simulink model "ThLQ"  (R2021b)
settings: Solver=VariableStepAuto  StartTime=0.0  StopTime=timeWaypoints(end)-0.2  RelTol=1e-3
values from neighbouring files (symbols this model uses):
  a = 0.27    [CompareGazeboSimulink.m]    (also in RobotModel.m)
  b = 0.31    [CompareGazeboSimulink.m]    (also in RobotModel.m)
  D = abs(a-b)    [RobotModel.m]
  distAng = 0    [RobotModel.m]
  distVel = 0    [RobotModel.m]
  fro = 0.02    [CompareGazeboSimulink.m]    (also in RobotModel.m)
  fsl = 0.8    [CompareGazeboSimulink.m]    (also in RobotModel.m)
  fsly = 0.8    [CompareGazeboSimulink.m]    (also in RobotModel.m)
  I = (1/12)*m*((2*t)^2 + 0.12^2) + 1.5    (= 2.384)    [CompareGazeboSimulink.m]    (also in RobotModel.m = 0.866666666667)
  k = 1    [RobotModel.m]
  ko = 0    [CompareGazeboSimulink.m]    (also in RobotModel.m = 0.25)
  kt = 0.58    [CompareGazeboSimulink.m]    (also in RobotModel.m)
  kx = 0.5    [RobotModel.m]
  ky = 0.5    [RobotModel.m]
  lx = 0.15    [RobotModel.m]
  ly = 0.15    [RobotModel.m]
  m = 51    [CompareGazeboSimulink.m]    (also in RobotModel.m = 50)
  mdy = 10    [CompareGazeboSimulink.m]    (also in RobotModel.m)
  mst = 10    [CompareGazeboSimulink.m]    (also in RobotModel.m)
  Q = [1 0    [RobotModel.m]
  r = 0.19    [CompareGazeboSimulink.m]    (also in RobotModel.m)
  R = [0.01 0    [RobotModel.m]
  T_vel_variance = 0.0005    [RobotModel.m]
  Th0 = 0    [CompareGazeboSimulink.m]    (also in RobotModel.m = 0.9714)
  Th_vel0 = 0    [CompareGazeboSimulink.m]    (also in RobotModel.m)
  timeWaypoints = [0, 3, 7.5, 10.5, 13.5, 18, 20.5]    [RobotModel.m]
  Ts = 0.01    [CompareGazeboSimulink.m]    (also in RobotModel.m = 0.05)
  waypoints = [0 5; 4 9; 8 1; 12 5; 8 9; 4 1; 0 5]    [CubicSpline.m]    (also in RobotModel.m = [0 2.5; 2 4.5; 4 0.5; 6 2.5; 4 4.5; 2 0.5; 0 2.5])
  X0 = 0    [CompareGazeboSimulink.m]    (also in RobotModel.m)
  x_vel0 = 0    [CompareGazeboSimulink.m]    (also in RobotModel.m)
  x_vel_variance = 0.0005    [RobotModel.m]
  Y0 = 0    [CompareGazeboSimulink.m]    (also in RobotModel.m = 2.5)
libraries: mobileRoboticsLib x1

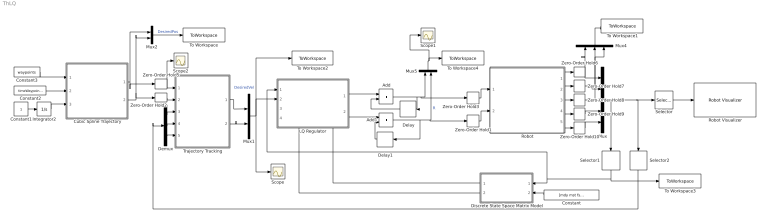
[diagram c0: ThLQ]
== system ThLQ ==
  Add : Sum
  Add1 : Sum
  Constant : Constant  Value=[mdy mst fsly r t a b m I Ts k]
  Constant1 : Constant
  Constant2 : Constant  Value=timeWaypoints
  Constant3 : Constant  Value=waypoints
  Cubic Spline Trajectory : MATLAB Function  TreatAsAtomicUnit=on
  Delay : Delay  DelayLength=1
  Delay1 : Delay  DelayLength=1
  Demux : Demux  Outputs=3
  Discrete State Space Matrix Model : MATLAB Function  TreatAsAtomicUnit=on
  Integrator2 : Integrator
  LQ Regulator : Subsystem
  Mux : Mux  Inputs=5
  Mux1 : Mux  Inputs=2
  Mux2 : Mux  Inputs=2
  Mux4 : Mux  Inputs=3
  Mux5 : Mux  Inputs=2
  Robot : Subsystem
  Robot Visualizer : mobileRoboticsLib/Environments/Robot Visualizer  Commented=on  robotRadius=0.3  showTrajectory=on  hasWaypoints=off  hasLidar=off  sensorOffset=[ 0, 0 ]  scanAngles=[ -pi/4, 0, pi/4 ]  hasObjDetector=off  objDetectorOffset=[ 0, 0 ]  objDetectorAngle=0  objDetectorFOV=pi/4  objDetectorMaxRange=5  objectColors=[ 1, 0, 0; 0, 1, 0; 0, 0, 1 ]  objectMarkers=s
  Scope : Scope
  Scope1 : Scope
  Scope2 : Scope
  Selector : Selector  InputPortWidth=5  IndexOptions=Index vector (dialog)  Indices=[1 2 3]  OutputSizes=1
  Selector1 : Selector  InputPortWidth=5  IndexOptions=Index vector (dialog)  Indices=[4 5]  OutputSizes=1
  Selector2 : Selector  InputPortWidth=5  IndexOptions=Index vector (dialog)  Indices=[1 2 3]  OutputSizes=1
  To Workspace : ToWorkspace  VariableName=desiredPos  SaveFormat=Timeseries  SampleTime=-1
  To Workspace1 : ToWorkspace  VariableName=ActualPos  SaveFormat=Timeseries  SampleTime=-1
  To Workspace2 : ToWorkspace  VariableName=DesiredVel  SaveFormat=Timeseries  SampleTime=-1
  To Workspace3 : ToWorkspace  VariableName=ActualVel  SaveFormat=Timeseries  SampleTime=-1
  To Workspace4 : ToWorkspace  VariableName=Forces  SaveFormat=Timeseries  SampleTime=-1
  Trajectory Tracking : Subsystem
  Zero-Order Hold{1..3,5..10} (9 alike) : ZeroOrderHold  SampleTime=Ts
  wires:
  Mux5/1 -> Scope1/1, To Workspace4/1
  Zero-Order Hold10/1 -> Mux/5
  Robot/1(X) -> Zero-Order Hold6/1
  Mux4/1 -> To Workspace1/1
  Robot/2(Y) -> Zero-Order Hold7/1
  Zero-Order Hold9/1 -> Mux/4
  Robot/5(v) -> Zero-Order Hold10/1
  Robot/3(Theta) -> Zero-Order Hold8/1
  Mux/1 -> Selector1/1, Selector2/1, Selector/1
  Zero-Order Hold8/1 -> Mux4/3, Mux/3
  Mux1/1 -> Scope/1, To Workspace2/1, LQ Regulator/2(Desired State)  "DesiredVel"
  Zero-Order Hold3/1 -> Robot/1(Left Force)
  Discrete State Space Matrix Model/2(B) -> LQ Regulator/3(B)
  Zero-Order Hold1/1 -> Robot/2(Right Force)
  Constant/1 -> Discrete State Space Matrix Model/2(param)
  Zero-Order Hold7/1 -> Mux4/2, Mux/2
  Selector1/1 -> LQ Regulator/1(Actual State), Discrete State Space Matrix Model/1(State), To Workspace3/1
  Delay1/1 -> Add1/2
  Delay/1 -> Add/2
  Add1/1 -> Zero-Order Hold1/1, Mux5/2, Delay1/1  "R"
  LQ Regulator/2(Right Force) -> Add1/1
  LQ Regulator/1(" Left Force") -> Add/1
  Add/1 -> Mux5/1, Zero-Order Hold3/1, Delay/1  "L"
  Robot/4(Theta') -> Zero-Order Hold9/1
  Discrete State Space Matrix Model/1(A) -> LQ Regulator/4(A)
  Selector/1 -> Robot Visualizer/1
  Cubic Spline Trajectory/1(X) -> Mux2/1, Zero-Order Hold5/1
  Constant3/1 -> Cubic Spline Trajectory/1(waypoints)
  Integrator2/1 -> Cubic Spline Trajectory/3(actualTime)
  Constant2/1 -> Cubic Spline Trajectory/2(time)
  Zero-Order Hold2/1 -> Trajectory Tracking/2(Yd)
  Mux2/1 -> To Workspace/1  "DesiredPos"
  Cubic Spline Trajectory/2(Y) -> Zero-Order Hold2/1, Mux2/2
  Constant1/1 -> Integrator2/1
  Zero-Order Hold5/1 -> Scope2/1, Trajectory Tracking/1(Xd)
  Trajectory Tracking/1(Angular Velocity) -> Mux1/1
  Trajectory Tracking/2(" Linear Velocity") -> Mux1/2
  Demux/1 -> Trajectory Tracking/3(X)
  Demux/2 -> Trajectory Tracking/4(Y)
  Demux/3 -> Trajectory Tracking/5(Theta)
  Selector2/1 -> Demux/1
  Zero-Order Hold6/1 -> Mux4/1, Mux/1

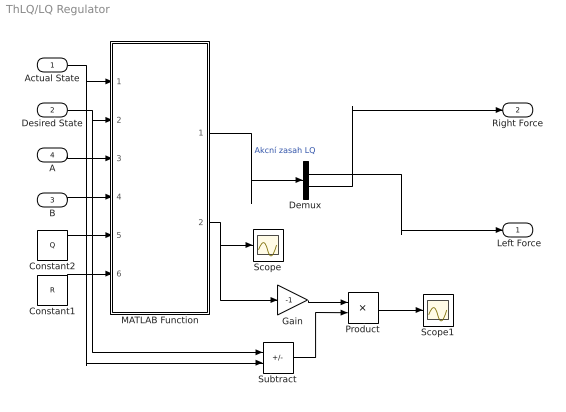
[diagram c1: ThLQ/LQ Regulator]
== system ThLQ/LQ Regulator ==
  Actual State : Inport
  Desired State : Inport  Port=2
  B : Inport  Port=3
  A : Inport  Port=4
  Constant1 : Constant  Value=R
  Constant2 : Constant  Value=Q
  Demux : Demux  Outputs=2
  Gain : Gain  Gain=-1
  MATLAB Function : MATLAB Function  TreatAsAtomicUnit=on
  Product : Product  Multiplication=Matrix(*)
  Scope : Scope
  Scope1 : Scope
  Subtract : Sum  Inputs=+-
  " Left Force" : Outport
  Right Force : Outport  Port=2
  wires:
  MATLAB Function/1(u) -> Demux/1  "Akcní zasah LQ"
  Actual State/1 -> Subtract/2, MATLAB Function/1(ActualState)
  Desired State/1 -> Subtract/1, MATLAB Function/2(DesiredState)
  A/1 -> MATLAB Function/3(A)
  B/1 -> MATLAB Function/4(B)
  Constant2/1 -> MATLAB Function/5(Q)
  Constant1/1 -> MATLAB Function/6(R)
  MATLAB Function/2(K) -> Gain/1, Scope/1
  Subtract/1 -> Product/2
  Gain/1 -> Product/1
  Product/1 -> Scope1/1
  Demux/1 -> " Left Force"/1
  Demux/2 -> Right Force/1

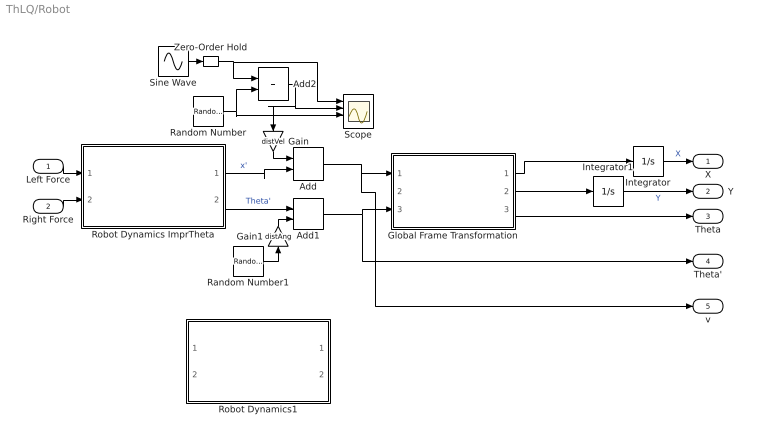
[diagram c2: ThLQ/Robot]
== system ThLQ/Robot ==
  Left Force : Inport
  Right Force : Inport  Port=2
  Add : Sum
  Add1 : Sum
  Add2 : Sum
  Gain : Gain  Gain=distVel
  Gain1 : Gain  Gain=distAng
  Global Frame Transformation : Subsystem
  Integrator : Integrator  InitialCondition=X0
  Integrator1 : Integrator  InitialCondition=Y0
  Random Number : RandomNumber  Variance=x_vel_variance  SampleTime=0.5
  Random Number1 : RandomNumber  Variance=T_vel_variance  SampleTime=0.1
  Robot Dynamics ImprTheta : Subsystem
  Robot Dynamics1 : Subsystem  Commented=on
  Scope : Scope  NumInputPorts=4
  Sine Wave : Sin  Amplitude=0.1  Frequency=0.2  SampleTime=0
  Zero-Order Hold : ZeroOrderHold  SampleTime=0.25
  X : Outport
  Y : Outport  Port=2
  Theta : Outport  Port=3
  Theta' : Outport  Port=4
  v : Outport  Port=5
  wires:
  Right Force/1 -> Robot Dynamics ImprTheta/2(Right Force)
  Global Frame Transformation/1(X') -> Integrator/1
  Integrator/1 -> X/1  "X"
  Left Force/1 -> Robot Dynamics ImprTheta/1(Left Force)
  Global Frame Transformation/2(Y') -> Integrator1/1
  Global Frame Transformation/3(Theta) -> Theta/1
  Integrator1/1 -> Y/1  "Y"
  Robot Dynamics ImprTheta/1(x') -> Add/2  "x'"
  Add/1 -> v/1, Global Frame Transformation/1(x')
  Robot Dynamics ImprTheta/2(Theta') -> Add1/1  "Theta'"
  Add1/1 -> Theta'/1, Global Frame Transformation/3(Theta')
  Random Number1/1 -> Gain1/1
  Random Number/1 -> Add2/2, Scope/3
  Add2/1 -> Gain/1, Scope/2
  Sine Wave/1 -> Zero-Order Hold/1
  Zero-Order Hold/1 -> Scope/1, Add2/1
  Gain/1 -> Add/1
  Gain1/1 -> Add1/2

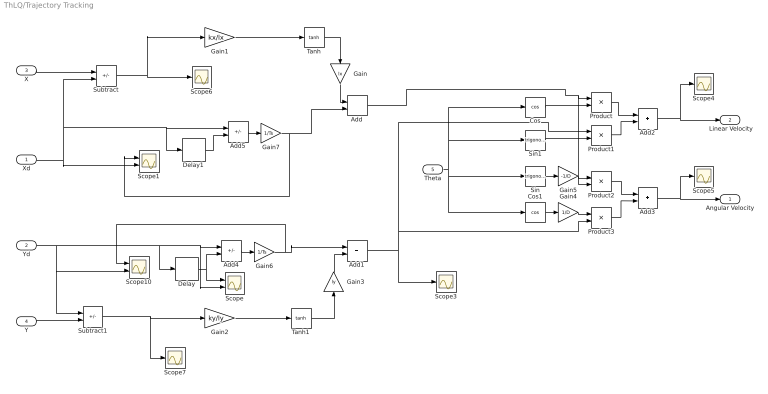
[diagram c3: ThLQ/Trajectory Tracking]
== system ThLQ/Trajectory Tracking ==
  Xd : Inport
  Yd : Inport  Port=2
  X : Inport  Port=3
  Y : Inport  Port=4
  Theta : Inport  Port=5
  Add{,1..3} (4 alike) : Sum
  Add4 : Sum  Inputs=+-
  Add5 : Sum  Inputs=+-
  Cos : Trigonometry  Operator=cos
  Cos1 : Trigonometry  Operator=cos
  Delay : Delay  DelayLength=1  InitialCondition=Y0
  Delay1 : Delay  DelayLength=1  InitialCondition=X0
  Gain : Gain  Gain=lx
  Gain1 : Gain  Gain=kx/lx
  Gain2 : Gain  Gain=ky/ly
  Gain3 : Gain  Gain=ly
  Gain4 : Gain  Gain=1/D
  Gain5 : Gain  Gain=-1/D
  Gain6 : Gain  Gain=1/Ts
  Gain7 : Gain  Gain=1/Ts
  Product{,1..3} (4 alike) : Product
  Scope : Scope  NumInputPorts=2
  Scope1 : Scope  NumInputPorts=2
  Scope10 : Scope  NumInputPorts=2
  Scope{3..7} (5 alike) : Scope
  Sin : Trigonometry
  Sin1 : Trigonometry
  Subtract : Sum  Inputs=-+
  Subtract1 : Sum  Inputs=+-
  Tanh : Trigonometry  Operator=tanh
  Tanh1 : Trigonometry  Operator=tanh
  Angular Velocity : Outport
  " Linear Velocity" : Outport  Port=2
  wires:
  Subtract/1 -> Gain1/1, Scope6/1
  Subtract1/1 -> Scope7/1, Gain2/1
  Add4/1 -> Gain6/1
  Tanh/1 -> Gain/1
  Gain1/1 -> Tanh/1
  Gain2/1 -> Tanh1/1
  Tanh1/1 -> Gain3/1
  Cos1/1 -> Gain4/1
  Sin/1 -> Gain5/1
  Theta/1 -> Cos/1, Sin1/1, Cos1/1, Sin/1
  Cos/1 -> Product/2
  Add/1 -> Product2/2, Product/1
  Sin1/1 -> Product1/2
  Gain5/1 -> Product2/1
  Gain4/1 -> Product3/1
  Add1/1 -> Scope3/1, Product3/2, Product1/1
  Product/1 -> Add2/1
  Product1/1 -> Add2/2
  Product2/1 -> Add3/1
  Product3/1 -> Add3/2
  Add2/1 -> Scope4/1, " Linear Velocity"/1
  Add3/1 -> Scope5/1, Angular Velocity/1
  Y/1 -> Subtract1/2
  Yd/1 -> Delay/1, Add4/1, Scope/2, Scope10/2, Subtract1/1
  X/1 -> Subtract/1
  Gain/1 -> Add/1
  Gain3/1 -> Add1/2
  Delay/1 -> Scope/1, Add4/2
  Gain6/1 -> Scope10/1, Add1/1
  Gain7/1 -> Scope1/1, Add/2
  Delay1/1 -> Add5/2
  Xd/1 -> Scope1/2, Delay1/1, Add5/1, Subtract/2
  Add5/1 -> Gain7/1

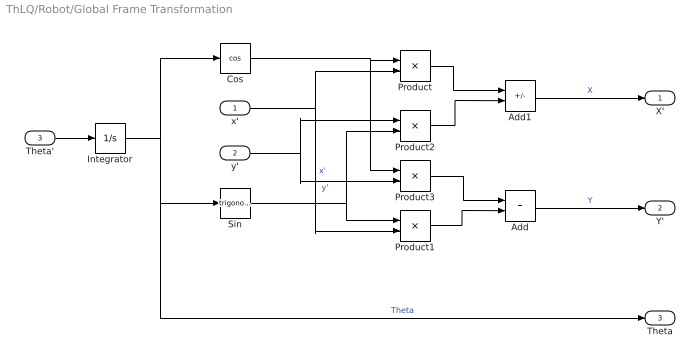
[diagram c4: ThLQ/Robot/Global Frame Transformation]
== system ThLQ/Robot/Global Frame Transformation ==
  x' : Inport
  y' : Inport  Port=2
  Theta' : Inport  Port=3
  Add : Sum
  Add1 : Sum  Inputs=+-
  Cos : Trigonometry  Operator=cos
  Integrator : Integrator  InitialCondition=Th0
  Product{,1..3} (4 alike) : Product
  Sin : Trigonometry
  X' : Outport
  Y' : Outport  Port=2
  Theta : Outport  Port=3
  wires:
  Add/1 -> Y'/1  "Y"
  Integrator/1 -> Theta/1, Sin/1, Cos/1  "Theta"
  Product1/1 -> Add/2
  x'/1 -> Product/2, Product1/2  "x'"
  Sin/1 -> Product1/1, Product2/2
  Product2/1 -> Add1/2
  Product3/1 -> Add/1
  Product/1 -> Add1/1
  Cos/1 -> Product/1, Product3/1
  y'/1 -> Product3/2, Product2/1  "y'"
  Add1/1 -> X'/1  "X"
  Theta'/1 -> Integrator/1

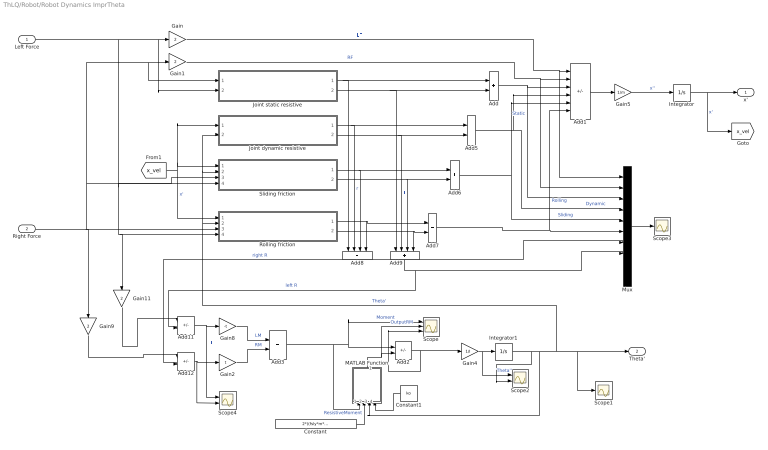
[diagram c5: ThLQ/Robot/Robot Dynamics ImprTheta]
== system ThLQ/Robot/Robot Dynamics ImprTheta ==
  Left Force : Inport
  Right Force : Inport  Port=2
  Add{,3,5..7} (5 alike) : Sum
  Add1 : Sum  Inputs=++----
  Add11 : Sum  Inputs=+-
  Add12 : Sum  Inputs=+-
  Add2 : Sum  Inputs=+-
  Add8 : Sum  Inputs=++++
  Add9 : Sum  Inputs=++++
  Constant : Constant  Value=2*((fsly*m*9.81)/(a+b))*a*b*kt
  Constant1 : Constant  Value=ko
  Gain{,1,9,11} (4 alike) : Gain  Gain=2
  Gain2 : Gain  Gain=t
  Gain4 : Gain  Gain=1/I
  Gain5 : Gain  Gain=1/m
  Gain8 : Gain  Gain=-t
  Integrator : Integrator  InitialCondition=x_vel0
  Integrator1 : Integrator  InitialCondition=Th_vel0
  Joint dynamic resistive : Subsystem
  Joint static resistive : Subsystem
  MATLAB Function : MATLAB Function  TreatAsAtomicUnit=on
  Mux : Mux  Inputs=10
  Rolling friction : Subsystem
  Scope : Scope  NumInputPorts=3
  Scope1 : Scope
  Scope2 : Scope  NumInputPorts=2
  Scope3 : Scope
  Scope4 : Scope  NumInputPorts=2
  Sliding friction : Subsystem
  x' : Outport
  Theta' : Outport  Port=2
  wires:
  Gain4/1 -> Scope2/1, Integrator1/1  "Theta''"
  Integrator1/1 -> Scope2/2, Sliding friction/2(Theta'), Joint dynamic resistive/2(Theta'), Rolling friction/2(Theta'), Scope1/1, Theta'/1, MATLAB Function/3(Omega)  "Theta'"
  Gain1/1 -> Mux/2, Add1/2  "RF"
  Add1/1 -> Gain5/1
  Gain5/1 -> Integrator/1  "x''"
  Integrator/1 -> x'/1, [x_vel]  "x'"
  [x_vel] -> Joint dynamic resistive/1("Local Long Velocity "), Sliding friction/1(Local longitudal velocity), Rolling friction/1(Local longitudal velocity)  "x'"
  Joint static resistive/2(Static Resistive Force Left) -> Add9/1, Add/2
  Joint dynamic resistive/1(Dynamic Resistive Force Right) -> Add8/2, Add5/1  "r"
  Joint dynamic resistive/2(Dynamic Resistive Force Left) -> Add9/2, Add5/2  "l"
  Sliding friction/1(Friction Right Force) -> Add8/3, Add6/1
  Sliding friction/2(Friction Left Force) -> Add9/3, Add6/2
  Rolling friction/1(Friction Right Force) -> Add8/4, Add7/1
  Rolling friction/2(Friction Left Force) -> Add9/4, Add7/2
  Add/1 -> Add1/3, Mux/3  "Static"
  Add6/1 -> Add1/5, Mux/5  "Sliding"
  Add7/1 -> Mux/6, Add1/6  "Rolling"
  Add5/1 -> Mux/4, Add1/4  "Dynamic"
  Add9/1 -> Add11/2, Mux/8  "left R"
  Add8/1 -> Add12/2, Mux/7  "right R"
  Mux/1 -> Scope3/1
  Add11/1 -> Scope4/1, Gain8/1  "LL"
  Add12/1 -> Scope4/2, Gain2/1
  Gain9/1 -> Add12/1
  Gain11/1 -> Add11/1
  Gain8/1 -> Add3/1  "LM"
  Gain2/1 -> Add3/2  "RM"
  Gain/1 -> Mux/1, Add1/1  "LF"
  Joint static resistive/1(Static Resistive Force Right) -> Add8/1, Add/1
  Add2/1 -> Scope/3, Gain4/1
  Add3/1 -> Scope/1, Add2/1, MATLAB Function/1(Moment)  "Moment"
  MATLAB Function/1(y) -> Scope/2, Add2/2  "OutputRM"
  Constant/1 -> MATLAB Function/2(ResistiveMoment)  "ResistiveMoment"
  Left Force/1 -> Gain11/1, Rolling friction/4(Fl), Sliding friction/4(Fl), Joint static resistive/2("Fl "), Gain/1
  Right Force/1 -> Gain9/1, Rolling friction/3(Fr), Sliding friction/3(Fr), Joint static resistive/1(Fr), Gain1/1
  Constant1/1 -> MATLAB Function/4(ko)

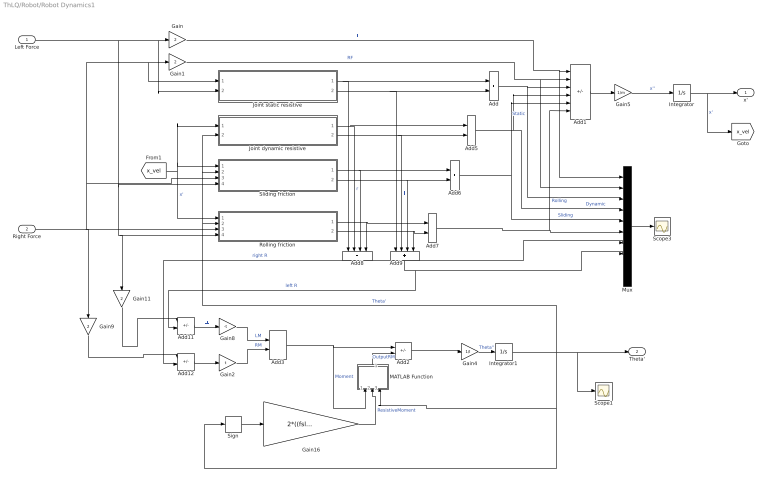
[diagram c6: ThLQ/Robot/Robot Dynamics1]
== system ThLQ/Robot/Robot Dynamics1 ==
  Left Force : Inport
  Right Force : Inport  Port=2
  Add{,3,5..7} (5 alike) : Sum
  Add1 : Sum  Inputs=++----
  Add11 : Sum  Inputs=+-
  Add12 : Sum  Inputs=+-
  Add2 : Sum  Inputs=+-
  Add8 : Sum  Inputs=++++
  Add9 : Sum  Inputs=++++
  Gain{,1,9,11} (4 alike) : Gain  Gain=2
  Gain16 : Gain  Gain=2*((fsly*m*9.81)/(a+b))*a*b
  Gain2 : Gain  Gain=t
  Gain4 : Gain  Gain=1/I
  Gain5 : Gain  Gain=1/m
  Gain8 : Gain  Gain=-t
  Integrator : Integrator  InitialCondition=x_vel0
  Integrator1 : Integrator  InitialCondition=Th_vel0
  Joint dynamic resistive : Subsystem
  Joint static resistive : Subsystem
  MATLAB Function : MATLAB Function  TreatAsAtomicUnit=on
  Mux : Mux  Inputs=10
  Rolling friction : Subsystem
  Scope1 : Scope
  Scope3 : Scope
  Sign : Signum
  Sliding friction : Subsystem
  x' : Outport
  Theta' : Outport  Port=2
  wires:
  Right Force/1 -> Rolling friction/3(Fr), Sliding friction/3(Fr), Joint static resistive/1(Fr), Gain1/1, Gain9/1
  Gain4/1 -> Integrator1/1  "Theta''"
  Integrator1/1 -> Sliding friction/2(Theta'), Joint dynamic resistive/2(Theta'), Rolling friction/2(Theta'), MATLAB Function/3(Omega), Sign/1, Scope1/1, Theta'/1  "Theta'"
  Left Force/1 -> Rolling friction/4(Fl), Gain11/1, Sliding friction/4(Fl), Joint static resistive/2("Fl "), Gain/1
  Gain1/1 -> Mux/2, Add1/2  "RF"
  Add1/1 -> Gain5/1
  Gain5/1 -> Integrator/1  "x''"
  Integrator/1 -> x'/1, [x_vel]  "x'"
  [x_vel] -> Joint dynamic resistive/1("Local Long Velocity "), Sliding friction/1(Local longitudal velocity), Rolling friction/1(Local longitudal velocity)  "x'"
  Joint static resistive/2(Static Resistive Force Left) -> Add9/1, Add/2
  Joint dynamic resistive/1(Dynamic Resistive Force Right) -> Add8/2, Add5/1  "r"
  Joint dynamic resistive/2(Dynamic Resistive Force Left) -> Add9/2, Add5/2  "l"
  Sliding friction/1(Friction Right Force) -> Add8/3, Add6/1
  Sliding friction/2(Friction Left Force) -> Add9/3, Add6/2
  Rolling friction/1(Friction Right Force) -> Add8/4, Add7/1
  Rolling friction/2(Friction Left Force) -> Add9/4, Add7/2
  Add/1 -> Add1/3, Mux/3  "Static"
  Add6/1 -> Add1/5, Mux/5  "Sliding"
  Add7/1 -> Mux/6, Add1/6  "Rolling"
  Add5/1 -> Mux/4, Add1/4  "Dynamic"
  Add9/1 -> Add11/2, Mux/8  "left R"
  Add8/1 -> Add12/2, Mux/7  "right R"
  Mux/1 -> Scope3/1
  Add11/1 -> Gain8/1  "LL"
  Add12/1 -> Gain2/1
  Gain9/1 -> Add12/1
  Gain11/1 -> Add11/1
  Gain8/1 -> Add3/1  "LM"
  Gain2/1 -> Add3/2  "RM"
  Gain/1 -> Mux/1, Add1/1  "LF"
  Joint static resistive/1(Static Resistive Force Right) -> Add8/1, Add/1
  Sign/1 -> Gain16/1
  Add2/1 -> Gain4/1
  Add3/1 -> Add2/1, MATLAB Function/1(Moment)  "Moment"
  MATLAB Function/1(y) -> Add2/2  "OutputRM"
  Gain16/1 -> MATLAB Function/2(ResistiveMoment)  "ResistiveMoment"

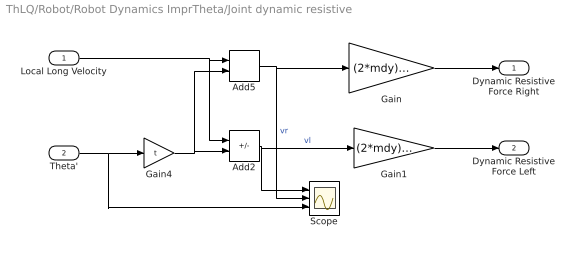
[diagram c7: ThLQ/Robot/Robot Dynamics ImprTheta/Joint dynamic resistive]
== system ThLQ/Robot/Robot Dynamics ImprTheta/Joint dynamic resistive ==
  "Local Long Velocity " : Inport
  Theta' : Inport  Port=2
  Add2 : Sum  Inputs=+-
  Add5 : Sum
  Gain : Gain  Gain=(2*mdy)/(r*r)
  Gain1 : Gain  Gain=(2*mdy)/(r*r)
  Gain4 : Gain  Gain=t
  Scope : Scope  NumInputPorts=3
  Dynamic Resistive Force Right : Outport
  Dynamic Resistive Force Left : Outport  Port=2
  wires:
  Gain/1 -> Dynamic Resistive Force Right/1
  Gain1/1 -> Dynamic Resistive Force Left/1
  Gain4/1 -> Add5/2, Add2/2
  Theta'/1 -> Scope/3, Gain4/1
  Add5/1 -> Scope/2, Gain/1  "vr"
  Add2/1 -> Scope/1, Gain1/1  "vl"
  "Local Long Velocity "/1 -> Add2/1, Add5/1

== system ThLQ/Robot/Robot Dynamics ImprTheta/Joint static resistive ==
  Fr : Inport
  "Fl " : Inport  Port=2
  Fsj : Gain  Gain=2*(mst/r)
  Fsj . : Gain  Gain=2*(mst/r)
  Gain1 : Gain  Gain=1/(mst/r)
  Gain2 : Gain  Gain=1/(mst/r)
  Tanh : Trigonometry  Operator=tanh
  Tanh1 : Trigonometry  Operator=tanh
  Static Resistive Force Right : Outport
  Static Resistive Force Left : Outport  Port=2
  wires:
  Fr/1 -> Gain1/1
  "Fl "/1 -> Gain2/1
  Tanh/1 -> Fsj/1
  Tanh1/1 -> Fsj ./1
  Gain1/1 -> Tanh/1
  Gain2/1 -> Tanh1/1
  Fsj/1 -> Static Resistive Force Right/1
  Fsj ./1 -> Static Resistive Force Left/1

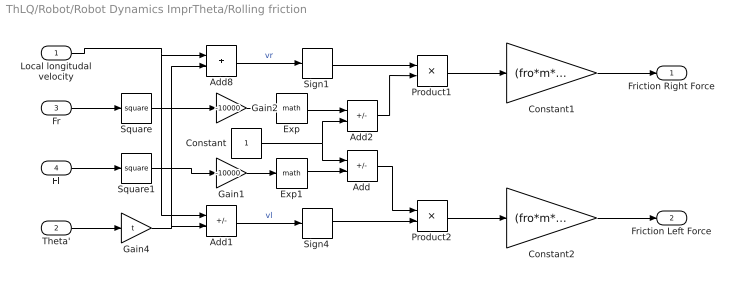
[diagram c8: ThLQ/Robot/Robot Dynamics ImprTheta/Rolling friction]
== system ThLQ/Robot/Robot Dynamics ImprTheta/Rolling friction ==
  Local longitudal velocity : Inport
  Theta' : Inport  Port=2
  Fr : Inport  Port=3
  Fl : Inport  Port=4
  Add : Sum  Inputs=+-
  Add1 : Sum  Inputs=+-
  Add2 : Sum  Inputs=-+
  Add8 : Sum
  Constant : Constant
  Constant1 : Gain  Gain=(fro*m*9.81)/2
  Constant2 : Gain  Gain=(fro*m*9.81)/2
  Exp : Math
  Exp1 : Math
  Gain1 : Gain  Gain=-10000
  Gain2 : Gain  Gain=-10000
  Gain4 : Gain  Gain=t
  Product1 : Product
  Product2 : Product
  Sign1 : Signum
  Sign4 : Signum
  Square : Math  Operator=square
  Square1 : Math  Operator=square
  Friction Right Force : Outport
  Friction Left Force : Outport  Port=2
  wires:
  Sign1/1 -> Product1/1
  Sign4/1 -> Product2/2
  Add8/1 -> Sign1/1  "vr"
  Fl/1 -> Square1/1
  Fr/1 -> Square/1
  Square1/1 -> Gain1/1
  Gain4/1 -> Add1/2, Add8/2
  Theta'/1 -> Gain4/1
  Add1/1 -> Sign4/1  "vl"
  Square/1 -> Gain2/1
  Gain2/1 -> Exp/1
  Gain1/1 -> Exp1/1
  Add2/1 -> Product1/2
  Add/1 -> Product2/1
  Exp1/1 -> Add/2
  Exp/1 -> Add2/1
  Constant/1 -> Add2/2, Add/1
  Local longitudal velocity/1 -> Add1/1, Add8/1
  Product1/1 -> Constant1/1
  Product2/1 -> Constant2/1
  Constant2/1 -> Friction Left Force/1
  Constant1/1 -> Friction Right Force/1

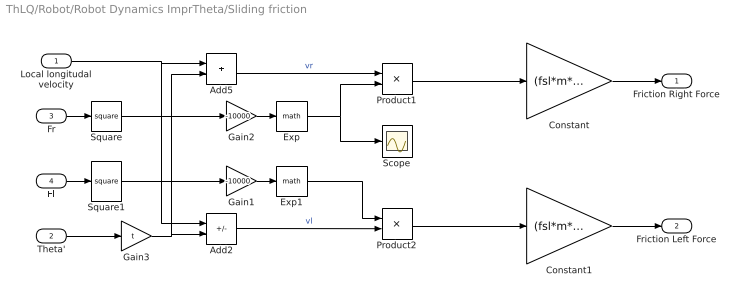
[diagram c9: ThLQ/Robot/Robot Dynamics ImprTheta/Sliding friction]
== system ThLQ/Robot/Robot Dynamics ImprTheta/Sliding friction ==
  Local longitudal velocity : Inport
  Theta' : Inport  Port=2
  Fr : Inport  Port=3
  Fl : Inport  Port=4
  Add2 : Sum  Inputs=+-
  Add5 : Sum
  Constant : Gain  Gain=(fsl*m*9.81)/2
  Constant1 : Gain  Gain=(fsl*m*9.81)/2
  Exp : Math
  Exp1 : Math
  Gain1 : Gain  Gain=-10000
  Gain2 : Gain  Gain=-10000
  Gain3 : Gain  Gain=t
  Product1 : Product
  Product2 : Product
  Scope : Scope
  Square : Math  Operator=square
  Square1 : Math  Operator=square
  Friction Right Force : Outport
  Friction Left Force : Outport  Port=2
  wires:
  Theta'/1 -> Gain3/1
  Gain3/1 -> Add2/2, Add5/2
  Add5/1 -> Product1/1  "vr"
  Add2/1 -> Product2/2  "vl"
  Exp/1 -> Scope/1, Product1/2
  Gain1/1 -> Exp1/1
  Gain2/1 -> Exp/1
  Fr/1 -> Square/1
  Fl/1 -> Square1/1
  Square/1 -> Gain2/1
  Square1/1 -> Gain1/1
  Product1/1 -> Constant/1
  Product2/1 -> Constant1/1
  Exp1/1 -> Product2/1
  Local longitudal velocity/1 -> Add2/1, Add5/1
  Constant/1 -> Friction Right Force/1
  Constant1/1 -> Friction Left Force/1

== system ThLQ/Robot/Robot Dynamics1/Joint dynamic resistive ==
  "Local Long Velocity " : Inport
  Theta' : Inport  Port=2
  Add2 : Sum  Inputs=+-
  Add5 : Sum
  Gain : Gain  Gain=(2*mdy)/(r*r)
  Gain1 : Gain  Gain=(2*mdy)/(r*r)
  Gain4 : Gain  Gain=t
  Scope : Scope  NumInputPorts=3
  Dynamic Resistive Force Right : Outport
  Dynamic Resistive Force Left : Outport  Port=2
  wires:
  Gain/1 -> Dynamic Resistive Force Right/1
  Gain1/1 -> Dynamic Resistive Force Left/1
  Gain4/1 -> Add5/2, Add2/2
  Theta'/1 -> Scope/3, Gain4/1
  Add5/1 -> Scope/2, Gain/1  "vr"
  Add2/1 -> Scope/1, Gain1/1  "vl"
  "Local Long Velocity "/1 -> Add2/1, Add5/1

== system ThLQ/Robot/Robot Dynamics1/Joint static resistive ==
  Fr : Inport
  "Fl " : Inport  Port=2
  Fsj : Gain  Gain=2*(mst/r)
  Fsj . : Gain  Gain=2*(mst/r)
  Gain1 : Gain  Gain=1/(mst/r)
  Gain2 : Gain  Gain=1/(mst/r)
  Tanh : Trigonometry  Operator=tanh
  Tanh1 : Trigonometry  Operator=tanh
  Static Resistive Force Right : Outport
  Static Resistive Force Left : Outport  Port=2
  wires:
  Fr/1 -> Gain1/1
  "Fl "/1 -> Gain2/1
  Tanh/1 -> Fsj/1
  Tanh1/1 -> Fsj ./1
  Gain1/1 -> Tanh/1
  Gain2/1 -> Tanh1/1
  Fsj/1 -> Static Resistive Force Right/1
  Fsj ./1 -> Static Resistive Force Left/1

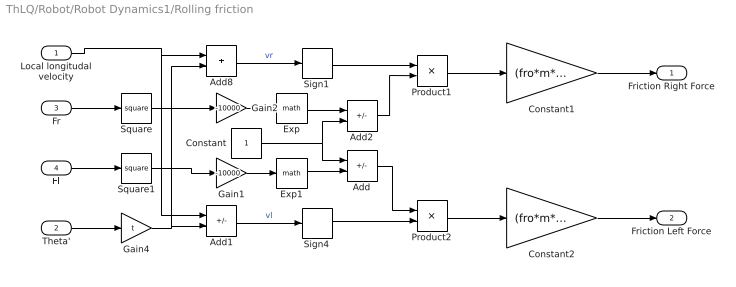
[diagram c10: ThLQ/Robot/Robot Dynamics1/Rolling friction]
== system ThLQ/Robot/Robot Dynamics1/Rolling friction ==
  Local longitudal velocity : Inport
  Theta' : Inport  Port=2
  Fr : Inport  Port=3
  Fl : Inport  Port=4
  Add : Sum  Inputs=+-
  Add1 : Sum  Inputs=+-
  Add2 : Sum  Inputs=-+
  Add8 : Sum
  Constant : Constant
  Constant1 : Gain  Gain=(fro*m*9.81)/2
  Constant2 : Gain  Gain=(fro*m*9.81)/2
  Exp : Math
  Exp1 : Math
  Gain1 : Gain  Gain=-10000
  Gain2 : Gain  Gain=-10000
  Gain4 : Gain  Gain=t
  Product1 : Product
  Product2 : Product
  Sign1 : Signum
  Sign4 : Signum
  Square : Math  Operator=square
  Square1 : Math  Operator=square
  Friction Right Force : Outport
  Friction Left Force : Outport  Port=2
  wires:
  Sign1/1 -> Product1/1
  Sign4/1 -> Product2/2
  Add8/1 -> Sign1/1  "vr"
  Fl/1 -> Square1/1
  Fr/1 -> Square/1
  Square1/1 -> Gain1/1
  Gain4/1 -> Add1/2, Add8/2
  Theta'/1 -> Gain4/1
  Add1/1 -> Sign4/1  "vl"
  Square/1 -> Gain2/1
  Gain2/1 -> Exp/1
  Gain1/1 -> Exp1/1
  Add2/1 -> Product1/2
  Add/1 -> Product2/1
  Exp1/1 -> Add/2
  Exp/1 -> Add2/1
  Constant/1 -> Add2/2, Add/1
  Local longitudal velocity/1 -> Add1/1, Add8/1
  Product1/1 -> Constant1/1
  Product2/1 -> Constant2/1
  Constant2/1 -> Friction Left Force/1
  Constant1/1 -> Friction Right Force/1

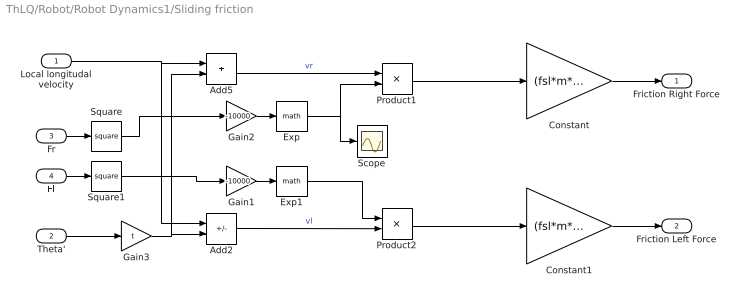
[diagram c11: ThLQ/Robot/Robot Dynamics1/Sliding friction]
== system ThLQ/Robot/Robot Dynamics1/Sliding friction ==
  Local longitudal velocity : Inport
  Theta' : Inport  Port=2
  Fr : Inport  Port=3
  Fl : Inport  Port=4
  Add2 : Sum  Inputs=+-
  Add5 : Sum
  Constant : Gain  Gain=(fsl*m*9.81)/2
  Constant1 : Gain  Gain=(fsl*m*9.81)/2
  Exp : Math
  Exp1 : Math
  Gain1 : Gain  Gain=-10000
  Gain2 : Gain  Gain=-10000
  Gain3 : Gain  Gain=t
  Product1 : Product
  Product2 : Product
  Scope : Scope
  Square : Math  Operator=square
  Square1 : Math  Operator=square
  Friction Right Force : Outport
  Friction Left Force : Outport  Port=2
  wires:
  Theta'/1 -> Gain3/1
  Gain3/1 -> Add2/2, Add5/2
  Add5/1 -> Product1/1  "vr"
  Add2/1 -> Product2/2  "vl"
  Exp/1 -> Scope/1, Product1/2
  Gain1/1 -> Exp1/1
  Gain2/1 -> Exp/1
  Fr/1 -> Square/1
  Fl/1 -> Square1/1
  Square/1 -> Gain2/1
  Square1/1 -> Gain1/1
  Product1/1 -> Constant/1
  Product2/1 -> Constant1/1
  Exp1/1 -> Product2/1
  Local longitudal velocity/1 -> Add2/1, Add5/1
  Constant/1 -> Friction Right Force/1
  Constant1/1 -> Friction Left Force/1

== matlab function ThLQ/Cubic Spline
Trajectory ==
function [X, Y] = TrajectoryGeneration(waypoints, time, actualTime)
%% Cubic spline
t = time;
Ax = zeros((size(waypoints,1)-1)*4);
Bx = zeros((size(waypoints,1)-1)*4, 1);

Ay = zeros((size(waypoints,1)-1)*4);
By = zeros((size(waypoints,1)-1)*4, 1);

%% Start and End Points (1-10)
% First polynom
Ax(1,1:4) = [t(1)^3 t(1)^2 t(1) 1];
Ax(2,1:4) = [t(2)^3 t(2)^2 t(2) 1];
Bx(1) = waypoints(1,1);
Bx(2) = waypoints(2,1);

Ay(1,1:4) = [t(1)^3 t(1)^2 t(1) 1];
Ay(2,1:4) = [t(2)^3 t(2)^2 t(2) 1];
By(1) = waypoints(1,2);
By(2) = waypoints(2,2);

% Second polynom
Ax(3,5:8) = [t(2)^3 t(2)^2 t(2) 1];
Ax(4,5:8) = [t(3)^3 t(3)^2 t(3) 1];
Bx(3) = waypoints(2,1);
Bx(4) = waypoints(3,1);

Ay(3,5:8) = [t(2)^3 t(2)^2 t(2) 1];
Ay(4,5:8) = [t(3)^3 t(3)^2 t(3) 1];
By(3) = waypoints(2,2);
By(4) = waypoints(3,2);

% Third polynom
Ax(5,9:12) = [t(3)^3 t(3)^2 t(3) 1];
Ax(6,9:12) = [t(4)^3 t(4)^2 t(4) 1];
Bx(5) = waypoints(3,1);
Bx(6) = waypoints(4,1);

Ay(5,9:12) = [t(3)^3 t(3)^2 t(3) 1];
Ay(6,9:12) = [t(4)^3 t(4)^2 t(4) 1];
By(5) = waypoints(3,2);
By(6) = waypoints(4,2);

% Fourth polynom
Ax(7,13:16) = [t(4)^3 t(4)^2 t(4) 1];
Ax(8,13:16) = [t(5)^3 t(5)^2 t(5) 1];
Bx(7) = waypoints(4,1);
Bx(8) = waypoints(5,1);

Ay(7,13:16) = [t(4)^3 t(4)^2 t(4) 1];
Ay(8,13:16) = [t(5)^3 t(5)^2 t(5) 1];
By(7) = waypoints(4,2);
By(8) = waypoints(5,2);

% Fifth polynom
Ax(9,17:20) = [t(5)^3 t(5)^2 t(5) 1];
Ax(10,17:20) = [t(6)^3 t(6)^2 t(6) 1];
Bx(9) = waypoints(5,1);
Bx(10) = waypoints(6,1);

Ay(9,17:20) = [t(5)^3 t(5)^2 t(5) 1];
Ay(10,17:20) = [t(6)^3 t(6)^2 t(6) 1];
By(9) = waypoints(5,2);
By(10) = waypoints(6,2);

% Sixth polynom
Ax(11,21:24) = [t(6)^3 t(6)^2 t(6) 1];
Ax(12,21:24) = [t(7)^3 t(7)^2 t(7) 1];
Bx(11) = waypoints(6,1);
Bx(12) = waypoints(7,1);

Ay(11,21:24) = [t(6)^3 t(6)^2 t(6) 1];
Ay(12,21:24) = [t(7)^3 t(7)^2 t(7) 1];
By(11) = waypoints(6,2);
By(12) = waypoints(7,2);

%% First derivation (11-14)
Ax(13, 1:8) = [3*t(2)^2 2*t(2) 1 0 -3*t(2)^2 -2*t(2) -1 0];
Ax(14, 5:12) = [3*t(3)^2 2*t(3) 1 0 -3*t(3)^2 -2*t(3) -1 0];
Ax(15, 9:16) = [3*t(4)^2 2*t(4) 1 0 -3*t(4)^2 -2*t(4) -1 0];
Ax(16, 13:20) = [3*t(5)^2 2*t(5) 1 0 -3*t(5)^2 -2*t(5) -1 0];
Ax(17, 17:24) = [3*t(6)^2 2*t(6) 1 0 -3*t(6)^2 -2*t(6) -1 0];

Ay(13, 1:8) = [3*t(2)^2 2*t(2) 1 0 -3*t(2)^2 -2*t(2) -1 0];
Ay(14, 5:12) = [3*t(3)^2 2*t(3) 1 0 -3*t(3)^2 -2*t(3) -1 0];
Ay(15, 9:16) = [3*t(4)^2 2*t(4) 1 0 -3*t(4)^2 -2*t(4) -1 0];
Ay(16, 13:20) = [3*t(5)^2 2*t(5) 1 0 -3*t(5)^2 -2*t(5) -1 0];
Ay(17, 17:24) = [3*t(6)^2 2*t(6) 1 0 -3*t(6)^2 -2*t(6) -1 0];

%% Second derivation (15-18)
Ax(18, 1:8) = [6*t(2) 2 0 0 -6*t(2) -2 0 0];
Ax(19, 5:12) = [6*t(3) 2 0 0 -6*t(3) -2 0 0];
Ax(20, 9:16) = [6*t(4) 2 0 0 -6*t(4) -2 0 0];
Ax(21, 13:20) = [6*t(5) 2 0 0 -6*t(5) -2 0 0];
Ax(22, 17:24) = [6*t(6) 2 0 0 -6*t(6) -2 0 0];

Ay(18, 1:8) = [6*t(2) 2 0 0 -6*t(2) -2 0 0];
Ay(19, 5:12) = [6*t(3) 2 0 0 -6*t(3) -2 0 0];
Ay(20, 9:16) = [6*t(4) 2 0 0 -6*t(4) -2 0 0];
Ay(21, 13:20) = [6*t(5) 2 0 0 -6*t(5) -2 0 0];
Ay(22, 17:24) = [6*t(6) 2 0 0 -6*t(6) -2 0 0];

%% Initial condition (19-20)
Ax(23, 1:4) = [3*t(1)^2 2*t(1) 1 0];
Ax(24, 21:24) = [3*t(end)^2 2*t(end) 1 0];
Bx(23) = 0;
Bx(24) = 0;

Ay(23, 1:4) = [3*t(1)^2 2*t(1) 1 0];
Ay(24, 21:24) = [3*t(end)^2 2*t(end) 1 0];
By(23) = 0;
By(24) = 0;

%% Solve equation
Px = Ax \ Bx;
Py = Ay \ By;

if(actualTime <= t(2))
    X = [actualTime^3 actualTime^2 actualTime 1]*Px(1:4);
    Y = [actualTime^3 actualTime^2 actualTime 1]*Py(1:4);
elseif(actualTime <= t(3))
    X = [actualTime^3 actualTime^2 actualTime 1]*Px(5:8);
    Y = [actualTime^3 actualTime^2 actualTime 1]*Py(5:8);
elseif(actualTime <= t(4))
    X = [actualTime^3 actualTime^2 actualTime 1]*Px(9:12);
    Y = [actualTime^3 actualTime^2 actualTime 1]*Py(9:12);
elseif(actualTime <= t(5))
    X = [actualTime^3 actualTime^2 actualTime 1]*Px(13:16);
    Y = [actualTime^3 actualTime^2 actualTime 1]*Py(13:16);
elseif(actualTime <= t(6))
    X = [actualTime^3 actualTime^2 actualTime 1]*Px(17:20);
    Y = [actualTime^3 actualTime^2 actualTime 1]*Py(17:20);
else
    X = [actualTime^3 actualTime^2 actualTime 1]*Px(21:24);
    Y = [actualTime^3 actualTime^2 actualTime 1]*Py(21:24);
end     


end

== matlab function ThLQ/Discrete State Space
Matrix Model ==
function [A, B] = fcn(State, param)  
    mdy = param(1);
    mst = param(2);
    fsly = param(3);
    r = param(4);
    t = param(5);
    a = param(6);
    b = param(7);
    m = param(8);
    I = param(9);
    Ts = param(10);
    k = param(11);
    
    O = State(1);
    
    A = eye(2) + [(-4*(mdy/(r*r))*t*t -2*(fsly*m*9.81/(a+b))*a*b)/I 0 ;
                  0 -4*(mdy/(r*r))/m]*Ts;

    % -2*(fsly*m*9.81/(a+b))*a*b*(2/3.14159)*(2/(1+2*2*O*O))
    B = Ts*[-2*t/I 2*t/I; 2/m 2/m];
end

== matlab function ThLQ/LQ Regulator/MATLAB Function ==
function [u, K]   = lq(ActualState, DesiredState, A, B, Q, R)                                                     

K_old = [ 0 0;
          0 0];
K     = [1 1;
         1 1];

% Co = ctrb(A,B); 
% unco = length(A) - rank(Co);

P = Q;
i = 0;
while (K ~= K_old)
    i = i + 1;
    K_old = K;
    P = Q + K'*R*K + (A - B*K)'*P*(A - B*K);
    K = (R + B'*P*B)^(-1)*B'*P*A;

    if (i > 100)
        break
    end
end

u = -K*(DesiredState - ActualState);
end

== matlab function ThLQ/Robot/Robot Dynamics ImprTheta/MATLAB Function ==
function y = fcn(Moment, ResistiveMoment, Omega, ko)
    y = Omega*ResistiveMoment;

%     if(abs(Moment) < abs(ResistiveMoment))
%         y = Moment;
%     else
%         y = (ko*Omega + sign(Omega))*ResistiveMoment;
%     end



end

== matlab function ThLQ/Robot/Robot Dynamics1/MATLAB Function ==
function y = fcn(Moment, ResistiveMoment, Omega)
    y = ResistiveMoment;
    
    if(Omega ~= 0)
        if(abs(Moment) < abs(ResistiveMoment))
            y = sign(Omega)*abs(Moment);
        else
            y = ResistiveMoment;
        end
    else
        y = 0;


end
